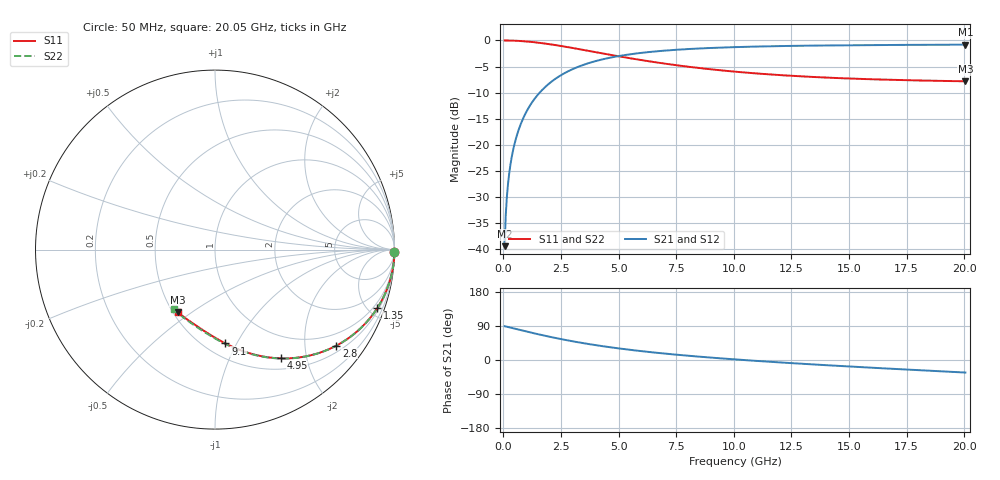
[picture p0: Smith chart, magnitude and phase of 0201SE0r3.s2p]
! AVX Thin Film Operation		Date: August 2001
! Description: Accu-P® Series, Thin Film, SMD, RF Capacitor
! Part Number: 02013J0R3ABW
! 50 MHz  -  20.05 GHz
! Serial Measurements
# mhz S db R 50
!	S11		S21		S12		S22
!	dB	Phase	dB	Phase	dB	Phase	dB	Phase
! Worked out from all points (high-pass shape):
!   401 points, 50 MHz to 20.05 GHz, reference 50 ohm
!   highest |S21| = -0.81 dB at 20.05 GHz (marker M1); lowest = -39.4 dB at 50 MHz (marker M2)
!   |S21| within 3 dB of the highest: 4.127 GHz to end of sweep
!   lowest |S11| = -7.8 dB at 20.05 GHz (marker M3), VSWR 2.37, Z = 26.4 - j22.1 ohm
!   |S11| at or under -10 dB: nowhere
!   |S22| runs from -7.9 to 0.0 dB; largest |S21 - S12| = 0
!   S11 on the Smith chart (normalised r, x): 50 MHz: open; 1.35 GHz: 0.66, -5.64; 2.8 GHz: 0.66, -2.74; 4.95 GHz: 0.65, -1.58; 9.1 GHz: 0.62, -0.90; 20.05 GHz: 0.53, -0.44
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50  -0.00 -0.8  -39.44 89.2  -39.44 89.2  -0.00 -0.8
100  -0.00 -1.5  -33.42 88.5  -33.42 88.5  -0.00 -1.5
200  -0.01 -3.0  -27.41 87.0  -27.41 87.0  -0.01 -3.0
250  -0.01 -3.8  -25.47 86.2  -25.47 86.2  -0.01 -3.8
350  -0.02 -5.3  -22.56 84.7  -22.56 84.7  -0.02 -5.3
450  -0.04 -6.8  -20.40 83.2  -20.40 83.2  -0.04 -6.8
600  -0.07 -9.0  -17.93 81.0  -17.93 81.0  -0.07 -9.0
800  -0.12 -11.9  -15.49 78.0  -15.49 78.0  -0.12 -11.9
1050  -0.21 -15.6  -13.23 74.4  -13.23 74.4  -0.21 -15.6
1350  -0.34 -19.8  -11.19 70.1  -11.19 70.1  -0.34 -19.8
2000  -0.71 -28.6  -8.20 61.4  -8.20 61.4  -0.71 -28.6
2800  -1.28 -38.3  -5.92 51.6  -5.92 51.6  -1.28 -38.3
3400  -1.76 -44.8  -4.79 45.1  -4.79 45.1  -1.76 -44.9
4100  -2.32 -51.6  -3.84 38.3  -3.84 38.3  -2.32 -51.7
4950  -3.00 -58.8  -3.03 31.0  -3.03 31.0  -3.00 -59.0
6750  -4.28 -71.3  -2.04 18.5  -2.04 18.5  -4.29 -71.6
7850  -4.94 -77.5  -1.69 12.2  -1.69 12.2  -4.95 -77.9
9100  -5.58 -83.6  -1.42 5.9  -1.42 5.9  -5.58 -84.3
10050  -5.98 -87.8  -1.28 1.6  -1.28 1.6  -5.99 -88.7
13400  -6.99 -100.5  -0.99 -11.6  -0.99 -11.6  -7.01 -102.1
16750  -7.54 -111.2  -0.86 -22.8  -0.86 -22.8  -7.56 -113.9
20050  -7.83 -120.8  -0.81 -33.1  -0.81 -33.1  -7.86 -124.7
